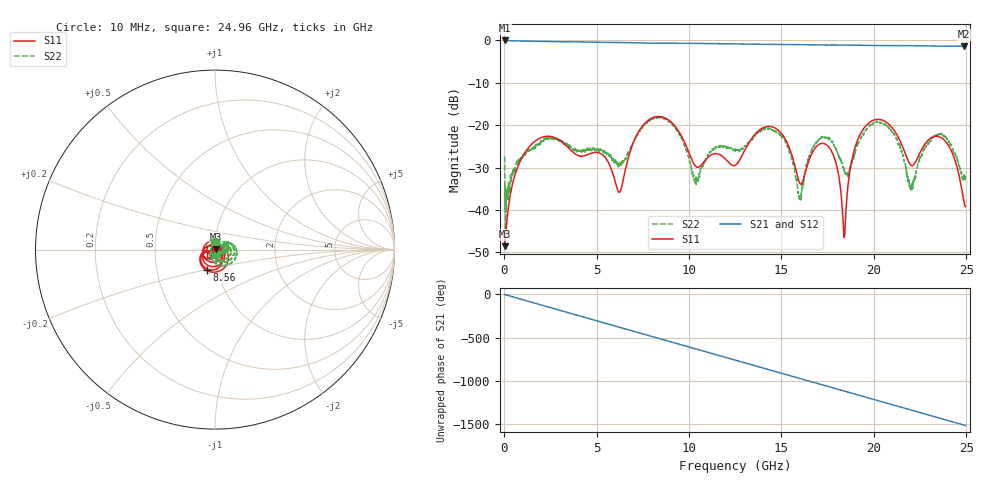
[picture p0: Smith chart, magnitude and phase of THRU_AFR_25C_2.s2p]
!Keysight Technologies,M9372A,MY54321388,A.12.55.09
!Automatic Fixture Removal (AFR)
!Date: Wednesday, May 22, 2019 8:33:21 AM
!S2P File: Measurements: S11,S21,S12,S22:
# MHz S  RI  R 50
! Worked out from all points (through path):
!   2496 points, 10 MHz to 24.96 GHz, reference 50 ohm
!   highest |S21| = -0.01 dB at 40 MHz (marker M1); lowest = -1.4 dB at 24.89 GHz (marker M2)
!   group delay of S21, straight-line fit = 168 ps
!   lowest |S11| = -48.5 dB at 20 MHz (marker M3), VSWR 1.01, Z = 50.3 + j0.139 ohm
!   |S11| at or under -10 dB: start of sweep to end of sweep
!   |S22| runs from -44.7 to -18.0 dB; largest |S21 - S12| = 1.4e-15
!   S11 on the Smith chart (normalised r, x): 10 MHz: 1.01, +0.00; 8.56 GHz: 0.89, -0.21; 24.96 GHz: 1.01, +0.02
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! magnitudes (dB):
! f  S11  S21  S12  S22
! 10 MHz  -46.9  -0.1  -0.1  -27.4
! 20 MHz  -48.5  0.0  0.0  -35.0
! 40 MHz  -47.9  0.0  0.0  -39.9
! 550 MHz  -32.0  -0.1  -0.1  -30.5
! 1.46 GHz  -24.5  -0.2  -0.2  -25.7
! 4.17 GHz  -27.3  -0.4  -0.4  -26.2
! 6.23 GHz  -35.8  -0.5  -0.5  -29.1
! 8.33 GHz  -18.0  -0.7  -0.7  -18.0
! 8.56 GHz  -18.1  -0.7  -0.7  -18.3
! 10.39 GHz  -29.8  -0.7  -0.7  -34.0
! 12.49 GHz  -29.5  -0.8  -0.8  -25.8
! 14.49 GHz  -20.4  -0.9  -0.9  -21.1
! 16 GHz  -33.8  -1.0  -1.0  -37.0
! 16.65 GHz  -26.6  -1.0  -1.0  -25.6
! 17.75 GHz  -26.5  -1.1  -1.1  -23.9
! 18.4 GHz  -46.5  -1.1  -1.1  -30.5
! 19.21 GHz  -22.6  -1.1  -1.1  -23.7
! 20.81 GHz  -19.8  -1.2  -1.2  -20.6
! 21.99 GHz  -29.4  -1.2  -1.2  -35.2
! 23.69 GHz  -23.1  -1.3  -1.3  -22.1
! 24.89 GHz  -38.3  -1.4  -1.4  -32.2
! 24.96 GHz  -39.2  -1.4  -1.4  -32.4
